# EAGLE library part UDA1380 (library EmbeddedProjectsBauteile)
Philips Stereo audio coder-decoder for MD, CD and MP3
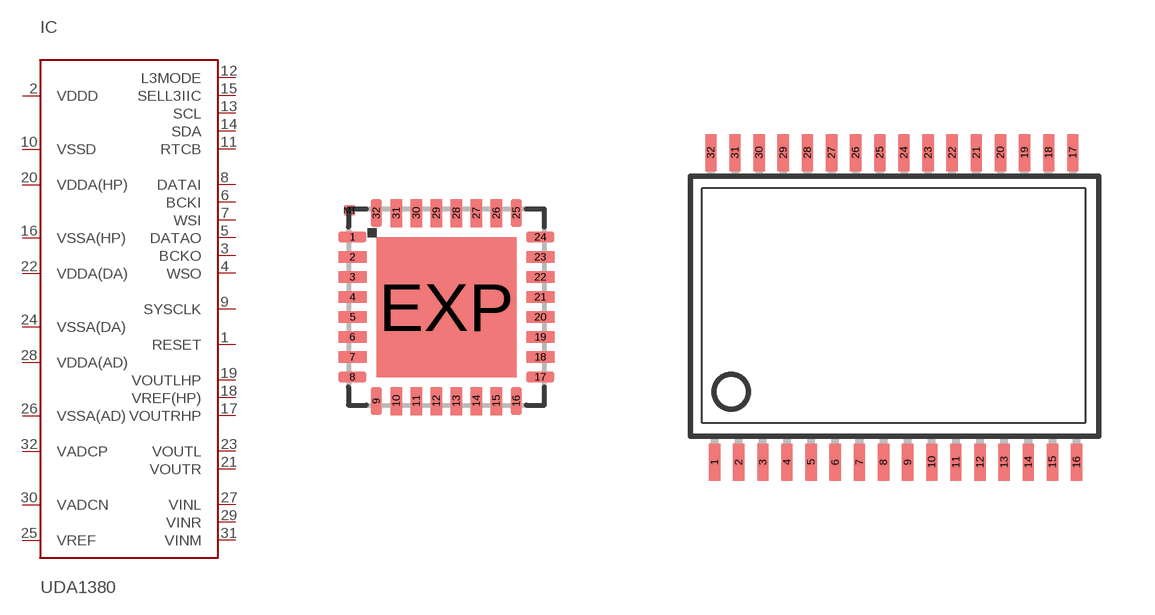
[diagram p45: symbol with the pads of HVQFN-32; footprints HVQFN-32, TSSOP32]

Designator prefix IC

## UDA1380HN  [HVQFN-32]
1  RESET  in
2  VDDD  pwr
3  BCKO  in
4  WSO  in
5  DATAO  in
6  BCKI  in
7  WSI  in
8  DATAI  in
9  SYSCLK  in
10  VSSD  pwr
11  RTCB  pwr
12  L3MODE  in
13  SCL
14  SDA
15  SELL3IIC  in
16  VSSA(HP)  pwr
17  VOUTRHP  out
18  VREF(HP)  in
19  VOUTLHP  out
20  VDDA(HP)  pwr
21  VOUTR  out
22  VDDA(DA)  pwr
23  VOUTL  out
24  VSSA(DA)  pwr
25  VREF  in
26  VSSA(AD)  pwr
27  VINL  in
28  VDDA(AD)  pwr
29  VINR  in
30  VADCN  pwr
31  VINM  in
32  VADCP  pwr

## UDA1380TT  [TSSOP32]
1  VINR  in
2  VADCN  pwr
3  VINM  in
4  VADCP  pwr
5  RESET  in
6  VDDD  pwr
7  BCKO  in
8  WSO  in
9  DATAO  in
10  BCKI  in
11  WSI  in
12  DATAI  in
13  SYSCLK  in
14  VSSD  pwr
15  RTCB  pwr
16  L3MODE  in
17  SCL
18  SDA
19  SELL3IIC  in
20  VSSA(HP)  pwr
21  VOUTRHP  out
22  VREF(HP)  in
23  VOUTLHP  out
24  VDDA(HP)  pwr
25  VOUTR  out
26  VDDA(DA)  pwr
27  VOUTL  out
28  VSSA(DA)  pwr
29  VREF  in
30  VSSA(AD)  pwr
31  VINL  in
32  VDDA(AD)  pwr

## Footprint HVQFN-32 (pad centres in mm)
smd 0.7 x 0.28: 1 -2.35,1.75; 2 -2.35,1.25; 3 -2.35,0.75; 4 -2.35,0.25; 5 -2.35,-0.25; 6 -2.35,-0.75; 7 -2.35,-1.25; 8 -2.35,-1.75; 17 2.35,-1.75; 18 2.35,-1.25; 19 2.35,-0.75; 20 2.35,-0.25; 21 2.35,0.25; 22 2.35,0.75; 23 2.35,1.25; 24 2.35,1.75
smd 0.28 x 0.7: 9 -1.75,-2.35; 10 -1.25,-2.35; 11 -0.75,-2.35; 12 -0.25,-2.35; 13 0.25,-2.35; 14 0.75,-2.35; 15 1.25,-2.35; 16 1.75,-2.35; 25 1.75,2.35; 26 1.25,2.35; 27 0.75,2.35; 28 0.25,2.35; 29 -0.25,2.35; 30 -0.75,2.35; 31 -1.25,2.35; 32 -1.75,2.35
smd 3.5 x 3.5: EXP 0,0
smd 0.25 x 0.25: M1 -2.415,2.415

## Footprint TSSOP32 (pad centres in mm)
smd 0.305 x 0.991: 1 -4.849,-4.202; 2 -4.199,-4.202; 3 -3.549,-4.202; 4 -2.899,-4.202; 5 -2.249,-4.202; 6 -1.599,-4.202; 7 -0.949,-4.202; 8 -0.299,-4.202; 9 0.351,-4.202; 10 1.001,-4.202; 11 1.651,-4.202; 12 2.301,-4.202; 13 2.951,-4.202; 14 3.601,-4.202; 15 4.251,-4.202; 16 4.901,-4.202; 17 4.801,4.134; 18 4.151,4.134; 19 3.501,4.134; 20 2.851,4.134; 21 2.201,4.134; 22 1.551,4.134; 23 0.901,4.134; 24 0.251,4.134; 25 -0.399,4.134; 26 -1.049,4.134; 27 -1.699,4.134; 28 -2.349,4.134; 29 -2.999,4.134; 30 -3.649,4.134; 31 -4.299,4.134; 32 -4.949,4.134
